FUNCTION_BLOCK FB_SignalHandling 
VAR_INPUT
	bInput		AT %I*	: BOOL;			// 输入信号
END_VAR
VAR_OUTPUT
	bOut		AT %Q* 	: BOOL;			// 输出信号
END_VAR
VAR
	bEnableLocal		: BOOL;			// 本地的输入变量
END_VAR

// =========================================================
;
// =========================================================

METHOD Enable
VAR_INPUT
	bEnable		: BOOL;
END_VAR
// =========================================================
// 将输入信号存储到本地

	bEnableLocal := bEnable;

// =========================================================
END_METHOD

METHOD SetOutput
VAR_INPUT
END_VAR
// =========================================================
	
bOut := bInput AND bEnableLocal;

// =========================================================
END_METHOD

END_FUNCTION_BLOCK
